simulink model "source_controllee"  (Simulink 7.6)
settings: Solver=ode23t  StartTime=0.0  StopTime=5  RelTol=1e-3
InitFcn:
  | clc
  | delete *.mat
StopFcn:
  | close all
  | load somme.mat
  | plot(x(1,:),x(2,:),x(1,:),x(3,:),x(1,:),x(4,:))
  | grid
  | title('Rampe, sinusoïde et signal somme')
  | xlabel('temps')
libraries: powerlib x4, simulink x1

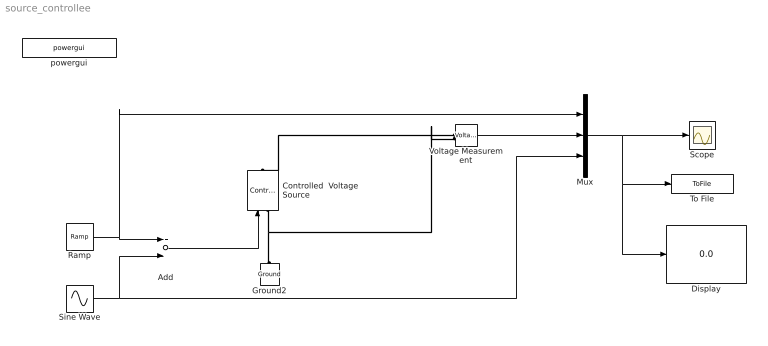
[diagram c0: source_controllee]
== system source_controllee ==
  Add : Sum
  Controlled  Voltage Source : powerlib/Electrical Sources/Controlled Voltage Source  DialogController=POWERSYS.PowerSysDialog  SystemSampleTime=-1  Initialize=on  Source_Type=AC  Amplitude=0  Phase=0  Frequency=0  Measurements=None
  Display : Display
  Ground2 : powerlib/Elements/Ground  DialogController=POWERSYS.PowerSysDialog  PhysicalDomain=powersysdomain  SubClassName=unknown  LeftPortType=p1  RightPortType=p1  LConnTagsString=a
  Mux : Mux  Inputs=3
  Ramp : simulink/Sources/Ramp  SystemSampleTime=-1  slope=1  start=0  X0=0
  Scope : Scope
  Sine Wave : Sin  Frequency=10  SampleTime=0
  To File : ToFile  Filename=somme  MatrixName=x
  Voltage Measurement : powerlib/Measurements/Voltage Measurement  DialogController=POWERSYS.PowerSysDialog  SystemSampleTime=-1  PhasorSimulation=off  OutputType=Complex  PSBequivalent=0
  powergui : powerlib/powergui  Priority=1  SystemSampleTime=-1  SimulationMode=Continuous  SampleTime=50e-6  frequency=60  SPID=off  DisableSnubberDevices=off  DisableRonSwitches=off  DisableVfSwitches=off  SwTol=0  Interpol=off  frequencyindice=0  echomessages=off  HookPort=off  DisplayEquations=off  FunctionMessages=off  EnableUseOfTLC=off  x0status=blocks  RestoreLinks=warning  ResistiveCurrentMeasurement=off  Ylog=off  Xlog=on  ShowGrid=off  save=off  variable=ZData  ZoomFFT=off  StartTime=0.0  cycles=1  DisplayStyle=1  fundamental=60  FreqAxis=off  MaxFrequency=1000  frequencyindicesteady=1  display=off  methode=off
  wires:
  Mux/1 -> Scope/1, To File/1, Display/1
  Sine Wave/1 -> Add/2, Mux/3
  Ramp/1 -> Add/1, Mux/1
  Add/1 -> Controlled  Voltage Source/1
  Voltage Measurement/1 -> Mux/2
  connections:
  Controlled  Voltage Source/LConn1 -- Ground2/LConn1 -- Voltage Measurement/LConn2
  Voltage Measurement/LConn1 -- Controlled  Voltage Source/RConn1
